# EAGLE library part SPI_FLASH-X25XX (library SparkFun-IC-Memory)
32M Serial Flash Memory 8pin SPI Flash series x25xx. Works with devices like W25X32 and BR25L32 Datasheet SparkFun Products SparkFun Venus GPS Logger (GPS-10920)
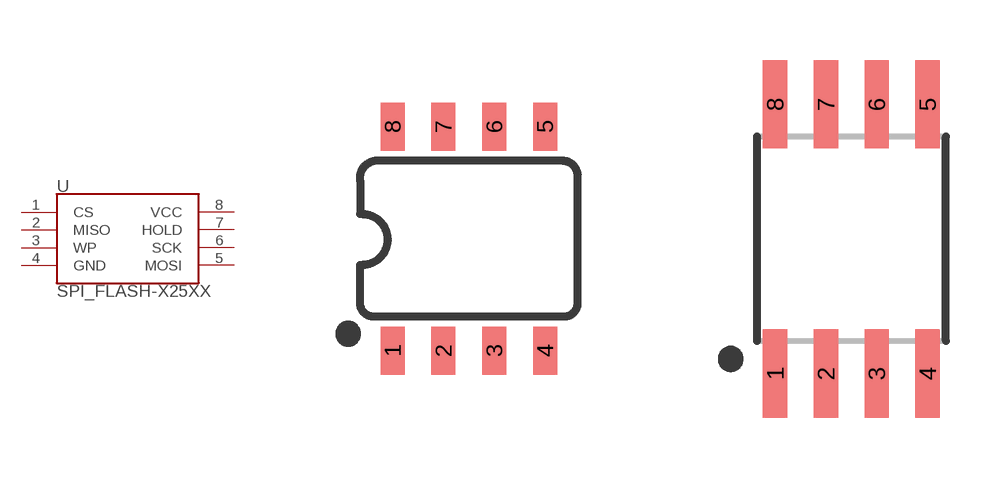
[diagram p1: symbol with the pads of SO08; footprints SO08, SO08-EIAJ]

Designator prefix U

## SPI_FLASH-X25XXSMD (PROD_ID: N/A; VALUE: 32M SPI Flash)  [SO08]
1  CS
2  MISO
3  WP
4  GND  pwr
5  MOSI
6  SCK
7  HOLD
8  VCC  pwr

## SPI_FLASH-X25XXSMD1 (PROD_ID: IC-09109; VALUE: 25F32006WSOI)  [SO08-EIAJ]
Pads as for SO08

## Footprint SO08 (pad centres in mm)
SOIC, 0.15 inch width
smd 0.6 x 1.2: 1 -1.905,-2.8; 2 -0.635,-2.8; 3 0.635,-2.8; 4 1.905,-2.8; 5 1.905,2.8; 6 0.635,2.8; 7 -0.635,2.8; 8 -1.905,2.8

## Footprint SO08-EIAJ (pad centres in mm)
Fits EIAJ packages (wide version of the SOIC-8).
smd 0.61 x 2.21: 1 -1.905,-3.378; 2 -0.635,-3.378; 3 0.635,-3.378; 4 1.905,-3.378; 5 1.905,3.353; 6 0.635,3.353; 7 -0.635,3.353; 8 -1.905,3.353

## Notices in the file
Licensing: Creative Commons ShareAlike 4.0 International - https://creativecommons.org/licenses/by-sa/4.0
